(* Logix 5000 Routine export FMSListProcessing; software revision 24.00 *)

TYPE FFLinkFMSResponse :
STRUCT
   Status : INT;   // 0=Success, 1=Timeout, 2=DLSeqMismatch, 3=InvokeIDMismatch, 4=FMSError
   DataLength : INT;
   CallBackID : DINT;
   Data : SINT[32];
END_STRUCT
END_TYPE

TYPE FFLinkFMSRequest :
STRUCT
   StationAddress : SINT;
   VFDSelector : SINT;   // 0=System, 1=AP
   Command : SINT;   // 0=Reserved, 1=Read, 2=Write
   CallBackID : DINT;
   TimeOut : INT;   // Timeout in milliseconds
   Index : INT;
   SubIndex : INT;
   DataLength : INT;
   Data : SINT[32];
END_STRUCT
END_TYPE

TYPE FFLinkFMSListItem :
STRUCT
   StationAddress : INT;   // H1 Device Station Address
   Command : INT;   // Command: 1=Read, 2=Write
   BlockIndex : INT;   // Object Index of Block
   Index : INT;   // Parameter Index
   SubIndex : INT;   // Parameter SubIndex (set to zero if n/a)
   DataType : INT;   // Parameter Data Type: 0=SINT, 1=INT, 2=DINT, 3=REAL
   ValueREAL : REAL;   // Parameter Value (R/W) when Data Type is REAL
   ValueDINT : DINT;   // Parameter Value (R/W) when Data Type is DINT
   ValueINT : INT;   // Parameter Value (R/W) when Data Type is INT
   ValueSINT : SINT;   // Parameter Value (R/W) when Data Type is SINT
   Status : INT;   // Status Integer returned by FF Link
   Busy : BOOL;   // Explciit Message Instruction Busy
   Success : BOOL;   // Transaction Succesful
   Fail : BOOL;   // Transaction Failed
   MsgError : BOOL;   // Explicit Message Failed (CIP / Connection Failure)
   DataLinkError : BOOL;   // Transaction failed due to H1 Data Link Error
   FMSError : BOOL;   // Transaction Failed due to FMS Error
   DataTypeError : BOOL;   // Transaction Failed due to Data Type / Size Inconsistency
   TimeOutError : BOOL;   // Transaction Failed due to Time-Out
   FMSErrorCode : DINT;   // The FMS Error Code (ErrorClass+ErrorCode) in the case of FMS Failure
END_STRUCT
END_TYPE

TYPE FFLinkFMSService :
STRUCT
   Request : FFLinkFMSRequest;
   Response : FFLinkFMSResponse;
END_STRUCT
END_TYPE

ADD_ON_INSTRUCTION FFLinkFMSGeneralRW   (* revision 1.0, vendor Aparian *)
VAR_INPUT
   StationAddress : INT; {required}
   Command : INT; {required}
   BlockIndex : INT; {required}
   Index : INT; {required}
   SubIndex : INT; {required}
   TimeOut : INT; {required}
   RequestDataLength : INT; {required}
   ResponseDataLength : INT; {required}
END_VAR
VAR_IN_OUT
   FMS : FFLinkFMSService; {required}
   Msg : MESSAGE; {required}
END_VAR
VAR_OUTPUT
   Busy : BOOL; {access Read Only, required}
   Success : BOOL; {access Read Only, required}
   Fail : BOOL; {access Read Only, required}
   MsgError : BOOL; {access Read Only, required}
   TimeOutErr : BOOL; {access Read Only, required}
   DataLinkErr : BOOL; {access Read Only, required}
   FMSError : BOOL; {access Read Only, required}
   Status : INT; {access Read Only, required}
   FMSErrorCode : DINT; {access Read Only, required}
   StatusOk : BOOL; {access Read Only, visible}
   ProcessData : BOOL; {visible}
END_VAR

ROUTINE Logic   (* ladder *)
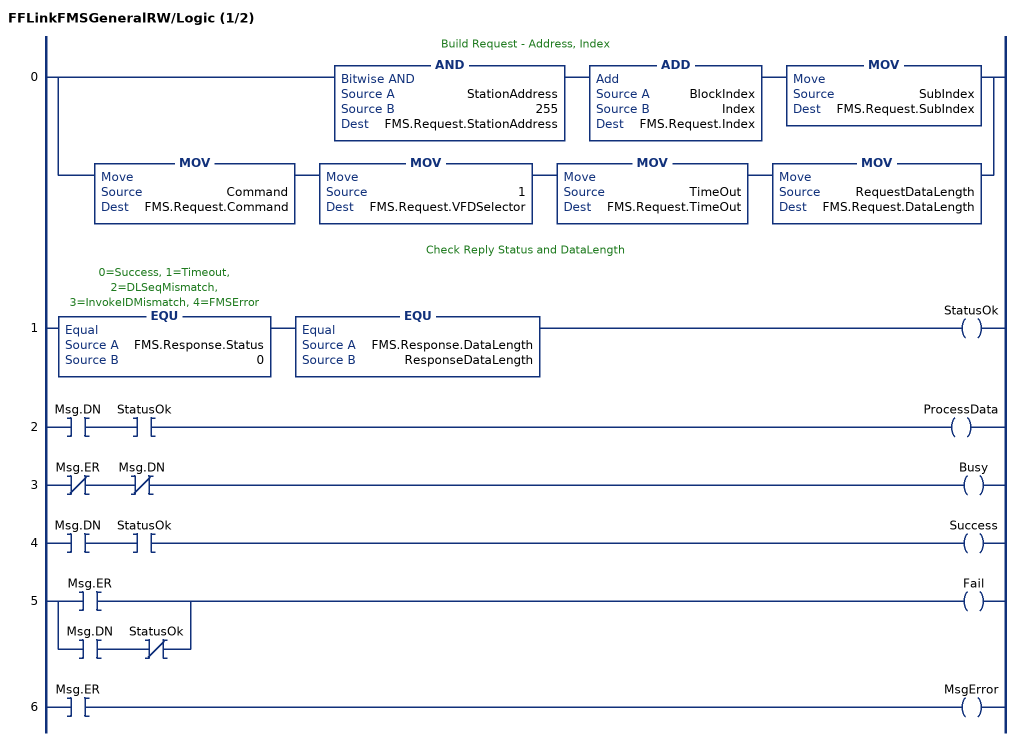
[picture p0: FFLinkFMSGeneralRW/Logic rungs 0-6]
   // Build Request - Address, Index
   0: [AND(StationAddress,255,FMS.Request.StationAddress) ADD(BlockIndex,Index,FMS.Request.Index) MOV(SubIndex,FMS.Request.SubIndex) ,MOV(Command,FMS.Request.Command) MOV(1,FMS.Request.VFDSelector) MOV(TimeOut,FMS.Request.TimeOut) MOV(RequestDataLength,FMS.Request.DataLength) ];
   // Check Reply Status and DataLength
   1: EQU(FMS.Response.Status,0)EQU(FMS.Response.DataLength,ResponseDataLength)OTE(StatusOk);
   2: XIC(Msg.DN)XIC(StatusOk)OTE(ProcessData);
   3: XIO(Msg.ER)XIO(Msg.DN)OTE(Busy);
   4: XIC(Msg.DN)XIC(StatusOk)OTE(Success);
   5: [XIC(Msg.ER) ,XIC(Msg.DN) XIO(StatusOk) ]OTE(Fail);
   6: XIC(Msg.ER)OTE(MsgError);
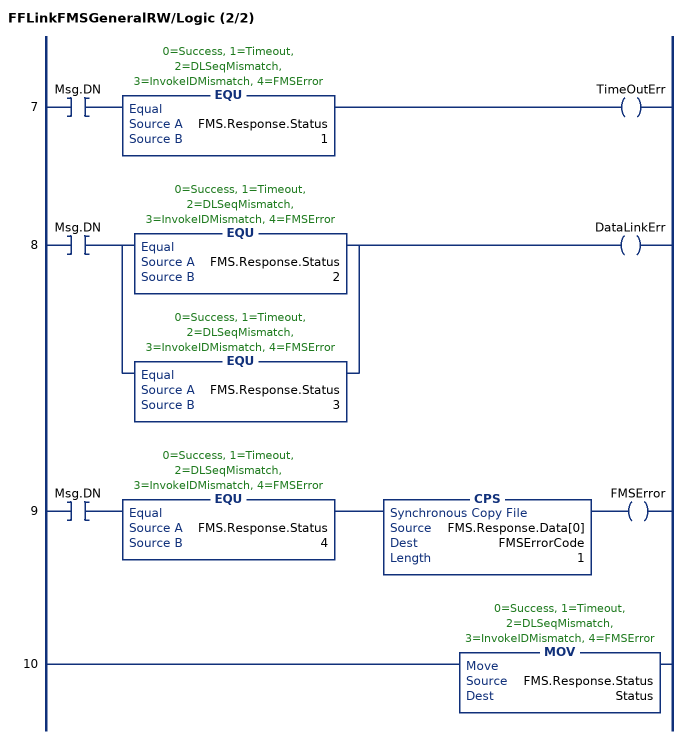
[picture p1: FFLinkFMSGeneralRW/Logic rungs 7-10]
   7: XIC(Msg.DN)EQU(FMS.Response.Status,1)OTE(TimeOutErr);
   8: XIC(Msg.DN)[EQU(FMS.Response.Status,2) ,EQU(FMS.Response.Status,3) ]OTE(DataLinkErr);
   9: XIC(Msg.DN)EQU(FMS.Response.Status,4)CPS(FMS.Response.Data[0],FMSErrorCode,1)OTE(FMSError);
   10: MOV(FMS.Response.Status,Status);
END_ROUTINE
END_ADD_ON_INSTRUCTION

ADD_ON_INSTRUCTION FFLinkListControl   (* revision 1.3, vendor Aparian *)
VAR_IN_OUT
   List : FFLinkFMSListItem[1]; {required}
END_VAR
VAR_INPUT
   MaximumItems : DINT; {required}
END_VAR
VAR_IN_OUT
   RequestIndex : INT; {required}
END_VAR
VAR_OUTPUT
   CurrentIndex : INT; {visible}
END_VAR
VAR_INPUT
   TimeOut : INT; {required}
END_VAR
VAR_OUTPUT
   MsgEnable : BOOL; {access Read Only}
END_VAR
VAR_IN_OUT
   FMS : FFLinkFMSService; {required}
   Msg : MESSAGE; {required}
END_VAR
VAR_OUTPUT
   Busy : BOOL; {access Read Only, visible}
END_VAR
VAR
   ProcessData : BOOL; {access None}
   LoadRequest : BOOL; {access None}
   Idx : DINT; {access None}
   TempINT : INT; {access None}
   TempDINT : DINT; {access None}
   TempREAL : REAL; {access None}
   GeneralRW : FFLinkFMSGeneralRW; {access None}
   PreviousIdx : DINT; {access None}
   BusyONS : BOOL; {access None}
   StatusOk : BOOL; {access None}
   DataSizeOk : BOOL; {access None}
   ScanCount : DINT; {access None}
   ProcessDataONS : BOOL; {access None}
   MessageFinishedONS : BOOL; {access None}
   MessageFinished : BOOL; {access None}
   TempDINT2 : DINT; {access None}
   DeadLockTimer : TIMER; {access None}
END_VAR

ROUTINE Logic   (* ladder *)
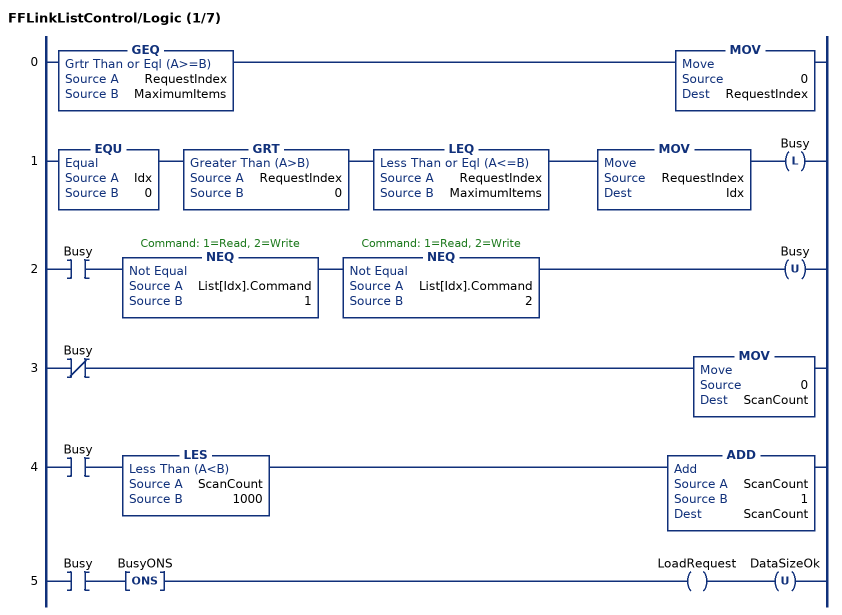
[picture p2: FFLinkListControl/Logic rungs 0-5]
   0: GEQ(RequestIndex,MaximumItems)MOV(0,RequestIndex);
   1: EQU(Idx,0)GRT(RequestIndex,0)LEQ(RequestIndex,MaximumItems)MOV(RequestIndex,Idx)OTL(Busy);
   2: XIC(Busy)NEQ(List[Idx].Command,1)NEQ(List[Idx].Command,2)OTU(Busy);
   3: XIO(Busy)MOV(0,ScanCount);
   4: XIC(Busy)LES(ScanCount,1000)ADD(ScanCount,1,ScanCount);
   5: XIC(Busy)ONS(BusyONS)OTE(LoadRequest)OTU(DataSizeOk);
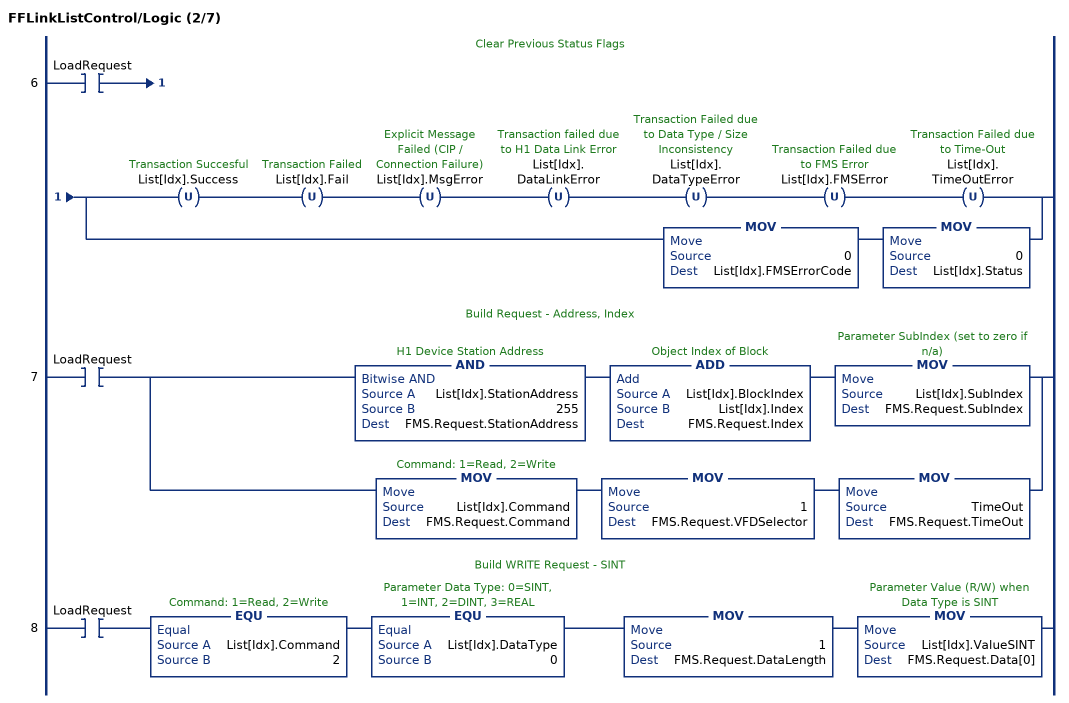
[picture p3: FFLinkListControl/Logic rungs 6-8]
   // Clear Previous Status Flags
   6: XIC(LoadRequest)[OTU(List[Idx].Success) OTU(List[Idx].Fail) OTU(List[Idx].MsgError) OTU(List[Idx].DataLinkError) OTU(List[Idx].DataTypeError) OTU(List[Idx].FMSError) OTU(List[Idx].TimeOutError) ,MOV(0,List[Idx].FMSErrorCode) MOV(0,List[Idx].Status) ];
   // Build Request - Address, Index
   7: XIC(LoadRequest)[AND(List[Idx].StationAddress,255,FMS.Request.StationAddress) ADD(List[Idx].BlockIndex,List[Idx].Index,FMS.Request.Index) MOV(List[Idx].SubIndex,FMS.Request.SubIndex) ,MOV(List[Idx].Command,FMS.Request.Command) MOV(1,FMS.Request.VFDSelector) MOV(TimeOut,FMS.Request.TimeOut) ];
   // Build WRITE Request - SINT
   8: XIC(LoadRequest)EQU(List[Idx].Command,2)EQU(List[Idx].DataType,0)MOV(1,FMS.Request.DataLength)MOV(List[Idx].ValueSINT,FMS.Request.Data[0]);
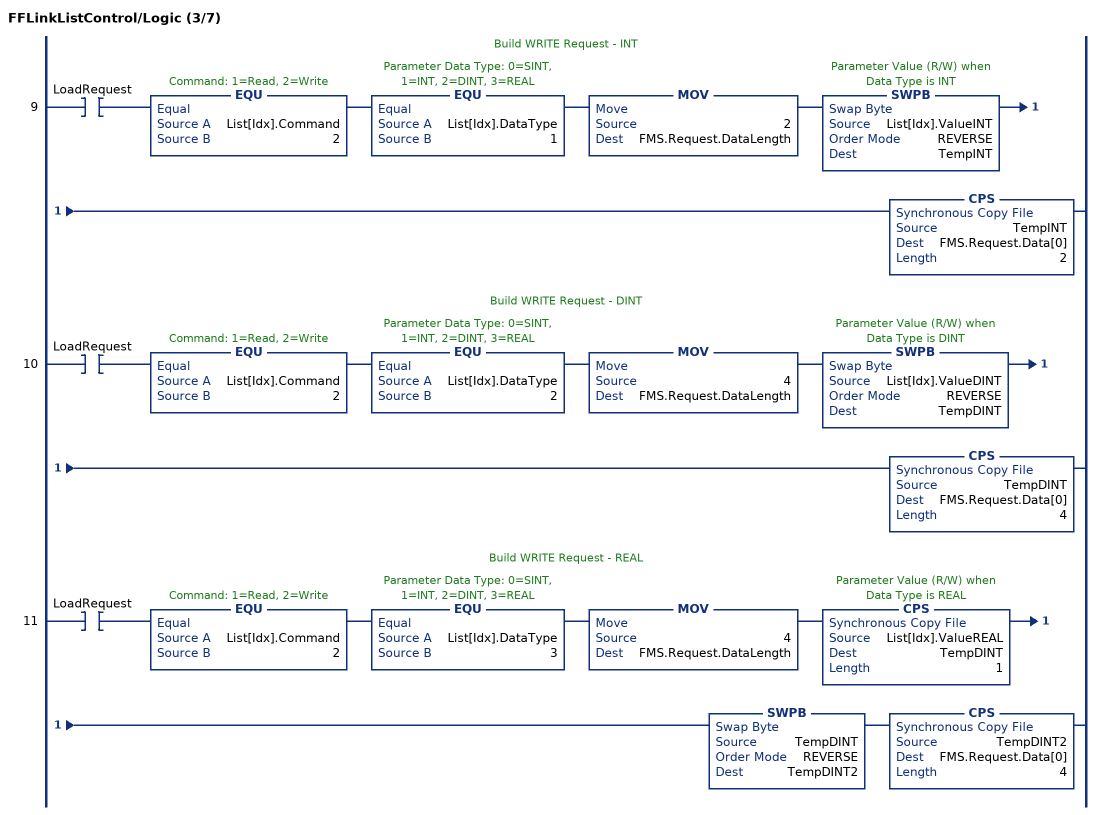
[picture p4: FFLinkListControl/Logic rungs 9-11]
   // Build WRITE Request - INT
   9: XIC(LoadRequest)EQU(List[Idx].Command,2)EQU(List[Idx].DataType,1)MOV(2,FMS.Request.DataLength)SWPB(List[Idx].ValueINT,REVERSE,TempINT)CPS(TempINT,FMS.Request.Data[0],2);
   // Build WRITE Request - DINT
   10: XIC(LoadRequest)EQU(List[Idx].Command,2)EQU(List[Idx].DataType,2)MOV(4,FMS.Request.DataLength)SWPB(List[Idx].ValueDINT,REVERSE,TempDINT)CPS(TempDINT,FMS.Request.Data[0],4);
   // Build WRITE Request - REAL
   11: XIC(LoadRequest)EQU(List[Idx].Command,2)EQU(List[Idx].DataType,3)MOV(4,FMS.Request.DataLength)CPS(List[Idx].ValueREAL,TempDINT,1)SWPB(TempDINT,REVERSE,TempDINT2)CPS(TempDINT2,FMS.Request.Data[0],4);
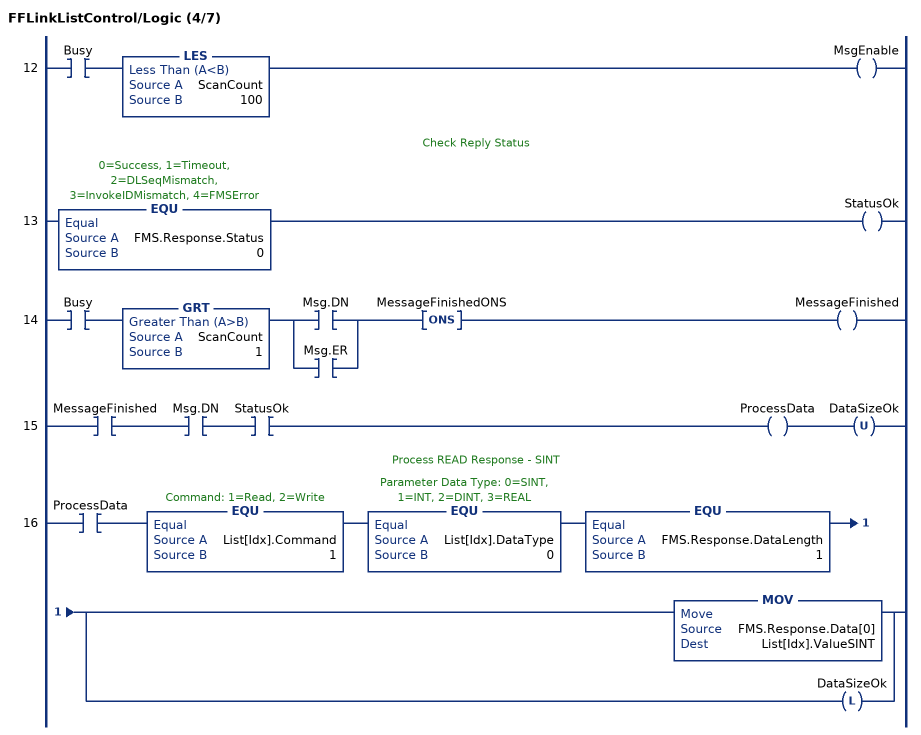
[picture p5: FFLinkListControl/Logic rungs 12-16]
   12: XIC(Busy)LES(ScanCount,100)OTE(MsgEnable);
   // Check Reply Status
   13: EQU(FMS.Response.Status,0)OTE(StatusOk);
   14: XIC(Busy)GRT(ScanCount,1)[XIC(Msg.DN) ,XIC(Msg.ER) ]ONS(MessageFinishedONS)OTE(MessageFinished);
   15: XIC(MessageFinished)XIC(Msg.DN)XIC(StatusOk)OTE(ProcessData)OTU(DataSizeOk);
   // Process READ Response - SINT
   16: XIC(ProcessData)EQU(List[Idx].Command,1)EQU(List[Idx].DataType,0)EQU(FMS.Response.DataLength,1)[MOV(FMS.Response.Data[0],List[Idx].ValueSINT) ,OTL(DataSizeOk) ];
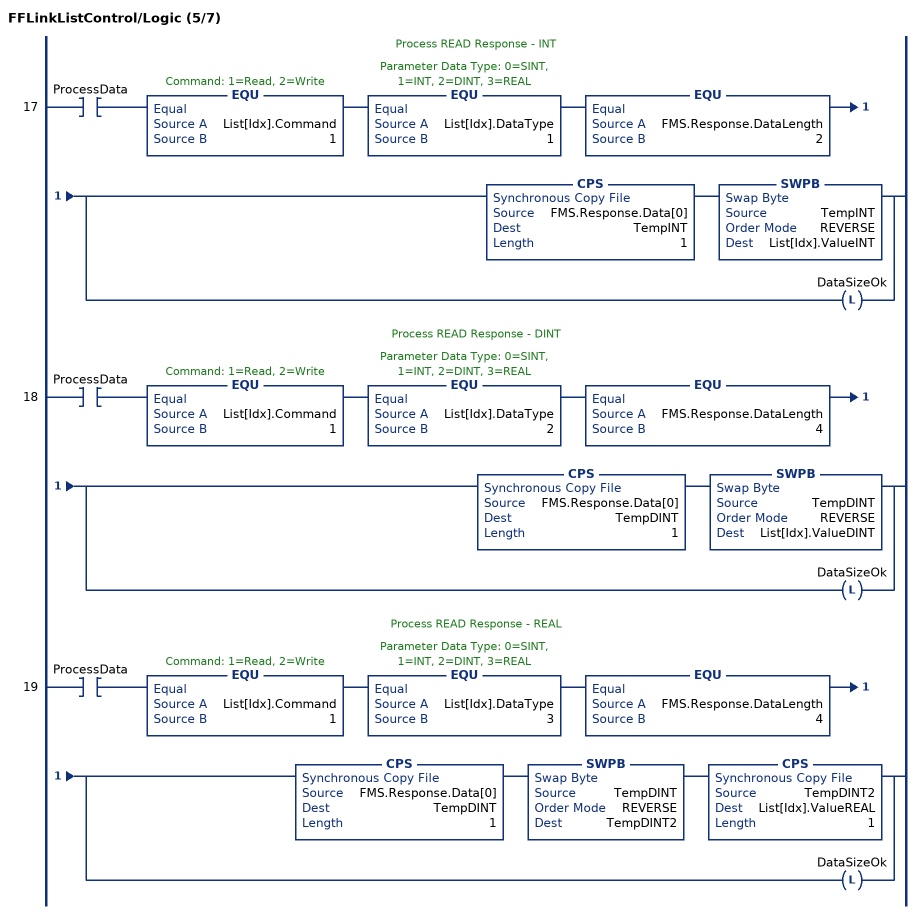
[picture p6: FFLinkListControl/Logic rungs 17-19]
   // Process READ Response - INT
   17: XIC(ProcessData)EQU(List[Idx].Command,1)EQU(List[Idx].DataType,1)EQU(FMS.Response.DataLength,2)[CPS(FMS.Response.Data[0],TempINT,1) SWPB(TempINT,REVERSE,List[Idx].ValueINT) ,OTL(DataSizeOk) ];
   // Process READ Response - DINT
   18: XIC(ProcessData)EQU(List[Idx].Command,1)EQU(List[Idx].DataType,2)EQU(FMS.Response.DataLength,4)[CPS(FMS.Response.Data[0],TempDINT,1) SWPB(TempDINT,REVERSE,List[Idx].ValueDINT) ,OTL(DataSizeOk) ];
   // Process READ Response - REAL
   19: XIC(ProcessData)EQU(List[Idx].Command,1)EQU(List[Idx].DataType,3)EQU(FMS.Response.DataLength,4)[CPS(FMS.Response.Data[0],TempDINT,1) SWPB(TempDINT,REVERSE,TempDINT2) CPS(TempDINT2,List[Idx].ValueREAL,1) ,OTL(DataSizeOk) ];
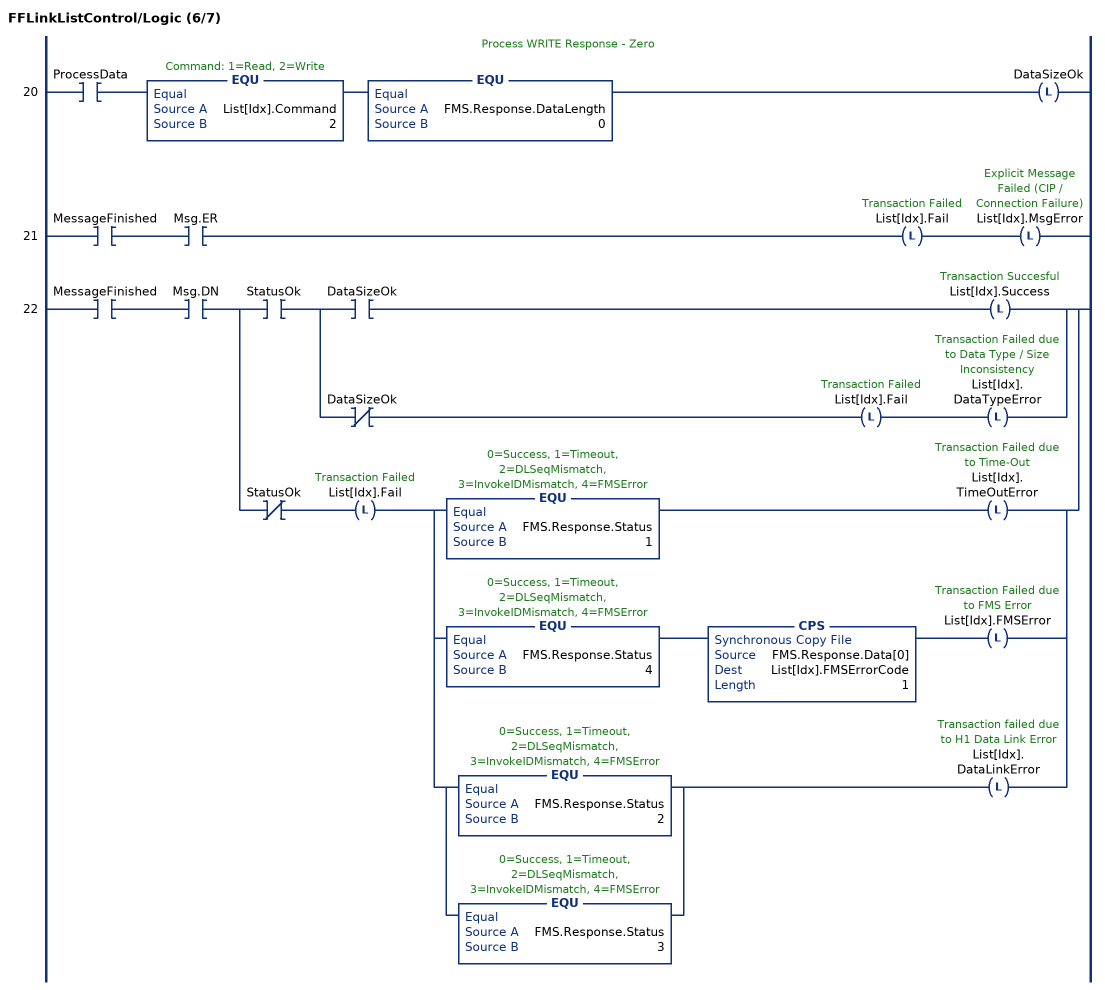
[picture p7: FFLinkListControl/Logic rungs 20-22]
   // Process WRITE Response - Zero
   20: XIC(ProcessData)EQU(List[Idx].Command,2)EQU(FMS.Response.DataLength,0)OTL(DataSizeOk);
   21: XIC(MessageFinished)XIC(Msg.ER)OTL(List[Idx].Fail)OTL(List[Idx].MsgError);
   22: XIC(MessageFinished)XIC(Msg.DN)[XIC(StatusOk) [XIC(DataSizeOk) OTL(List[Idx].Success) ,XIO(DataSizeOk) OTL(List[Idx].Fail) OTL(List[Idx].DataTypeError) ] ,XIO(StatusOk) OTL(List[Idx].Fail) [EQU(FMS.Response.Status,1) OTL(List[Idx].TimeOutError) ,EQU(FMS.Response.Status,4) CPS(FMS.Response.Data[0],List[Idx].FMSErrorCode,1) OTL(List[Idx].FMSError) ,[EQU(FMS.Response.Status,2) ,EQU(FMS.Response.Status,3) ] OTL(List[Idx].DataLinkError) ] ];
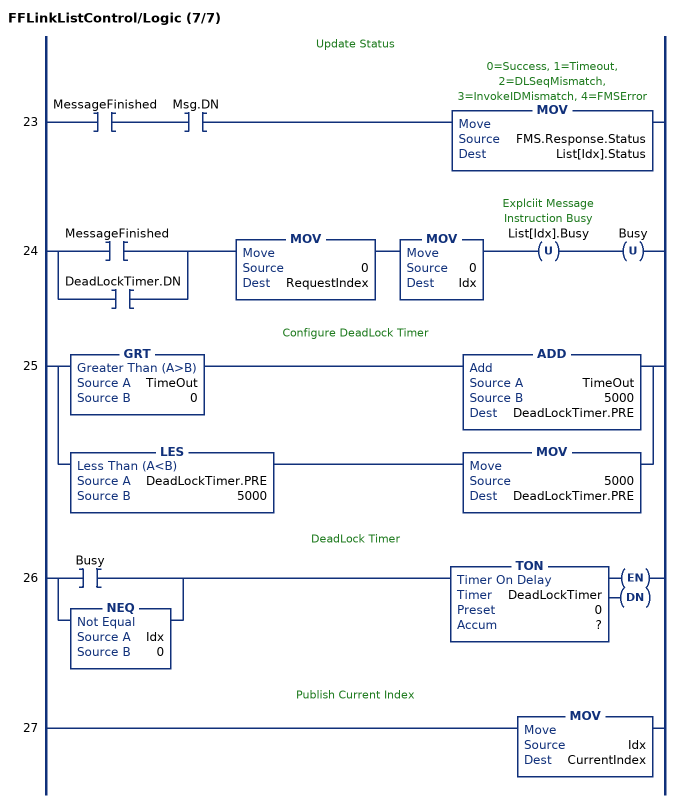
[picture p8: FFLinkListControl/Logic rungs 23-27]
   // Update Status
   23: XIC(MessageFinished)XIC(Msg.DN)MOV(FMS.Response.Status,List[Idx].Status);
   24: [XIC(MessageFinished) ,XIC(DeadLockTimer.DN) ]MOV(0,RequestIndex)MOV(0,Idx)OTU(List[Idx].Busy)OTU(Busy);
   // Configure DeadLock Timer
   25: [GRT(TimeOut,0) ADD(TimeOut,5000,DeadLockTimer.PRE) ,LES(DeadLockTimer.PRE,5000) MOV(5000,DeadLockTimer.PRE) ];
   // DeadLock Timer
   26: [XIC(Busy) ,NEQ(Idx,0) ]TON(DeadLockTimer,?,?);
   // Publish Current Index
   27: MOV(Idx,CurrentIndex);
END_ROUTINE
END_ADD_ON_INSTRUCTION

VAR_GLOBAL   (* controller tags *)
   FMSListControl01 : FFLinkListControl := (MaximumItems := 30, TimeOut := 2000);
   FMSMsg01 : MESSAGE;
        MessageParameters(MessageType := CIP Generic, RequestedLength := 32, ConnectedFlag := 2, ConnectionPath := FFL01, ServiceCode := 16#0066, ObjectType := 16#0434, TargetObject := 1, LocalElement := FMS01.Request, DestinationTag := FMS01.Response)
   FMSList01 : FFLinkFMSListItem[40];
   HMIFMSRequest : INT;
   FMS01 : FFLinkFMSService := (Request.StationAddress := 17, Request.VFDSelector := 1, Request.Command := 2, Request.TimeOut := 2000, Request.Index := 508, Request.SubIndex := 8, Request.DataLength := 4, Request.Data[0] := 65, Request.Data[1] := -8, Response.Data[0] := -127, Response.Data[1] := 97, Response.Data[2] := 7, Response.Data[3] := 18);
END_VAR

PROGRAM MainProgram

ROUTINE FMSListProcessing   (* ladder *)
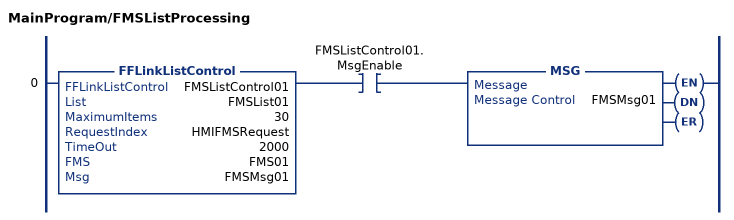
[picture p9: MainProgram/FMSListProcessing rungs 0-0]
   0: FFLinkListControl(FMSListControl01,FMSList01,30,HMIFMSRequest,2000,FMS01,FMSMsg01)XIC(FMSListControl01.MsgEnable)MSG(FMSMsg01);
END_ROUTINE
END_PROGRAM
